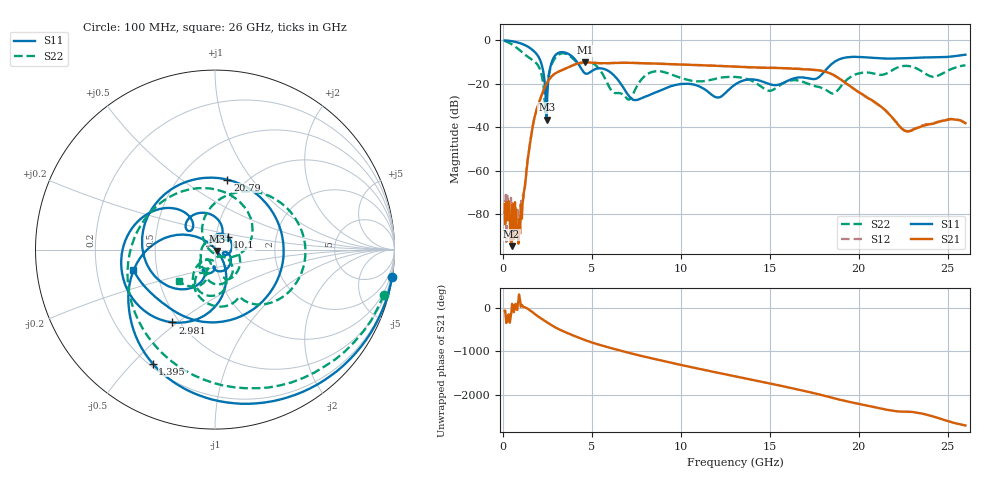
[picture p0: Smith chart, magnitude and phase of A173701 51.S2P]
!  2-Port S-parameters saved by WinCal
! VAR MeasName=S-Parameters (CALIBRATED_DATA) read from VNA (N5245A)
! VAR MeasDate=2017-6-7 10:31:49
! VAR NAME=A173701 51
! VAR FILENAME=A173701 51.S2P
! VAR DATE=2017-6-7 10:31:49
! VAR PHYS_PORTS=1,2
# Hz S DB R 50
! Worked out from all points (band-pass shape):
!   801 points, 100 MHz to 26 GHz, reference 50 ohm
!   highest |S21| = -10.10 dB at 4.633 GHz (marker M1); lowest = -94.9 dB at 488.5 MHz (marker M2)
!   |S21| within 3 dB of the highest: 3.48 GHz to 16.54 GHz (13.06 GHz wide, 130 % of centre); 16.64109 GHz to 16.64492 GHz (3.828 MHz wide, 0.023 % of centre)
!   lowest |S11| = -36.5 dB at 2.463 GHz (marker M3), VSWR 1.03, Z = 51.3 - j0.85 ohm
!   |S11| at or under -10 dB: 2.139 GHz to 2.749 GHz (610.1 MHz wide, 25 % of centre); 4.174 GHz to 18.62 GHz (14.45 GHz wide, 127 % of centre)
!   |S22| runs from -33.2 to -0.2 dB; largest |S21 - S12| = 0.0036
!   S11 on the Smith chart (normalised r, x): 100 MHz: 0, -13; 1.395 GHz: 0.21, -0.57; 2.981 GHz: 0.46, -0.48; 10.1 GHz: 1.14, +0.16; 20.79 GHz: 0.83, +0.77; 26 GHz: 0.37, -0.11
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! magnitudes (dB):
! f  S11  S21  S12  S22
! 100 MHz  0.0  -75.6  -80.2  -0.2
! 488.5 MHz  -0.3  -94.9  -76.1  -1.7
! 1.006 GHz  -1.4  -75.6  -79.3  -4.9
! 1.395 GHz  -2.8  -55.0  -55.2  -7.5
! 2.075 GHz  -8.7  -27.6  -27.6  -13.0
! 2.463 GHz  -36.5  -19.9  -19.9  -24.0
! 2.981 GHz  -6.6  -15.0  -15.0  -7.7
! 4.438 GHz  -13.4  -10.2  -10.2  -10.5
! 4.633 GHz  -15.2  -10.1  -10.1  -10.0
! 5.863 GHz  -13.7  -10.5  -10.5  -19.5
! 7.061 GHz  -25.3  -10.3  -10.3  -27.3
! 8.744 GHz  -23.4  -10.7  -10.7  -14.2
! 10.1 GHz  -20.0  -11.1  -11.1  -17.6
! 12.08 GHz  -26.3  -11.7  -11.7  -17.4
! 13.05 GHz  -20.4  -12.1  -12.0  -16.8
! 17.39 GHz  -17.8  -13.5  -13.5  -20.7
! 18.59 GHz  -10.2  -16.0  -15.9  -24.4
! 20.79 GHz  -8.0  -27.7  -28.0  -15.1
! 21.69 GHz  -8.4  -33.9  -33.9  -14.7
! 22.73 GHz  -8.2  -41.9  -41.8  -11.7
! 24.22 GHz  -7.8  -38.2  -38.1  -16.8
! 26 GHz  -6.6  -38.2  -38.0  -11.5
